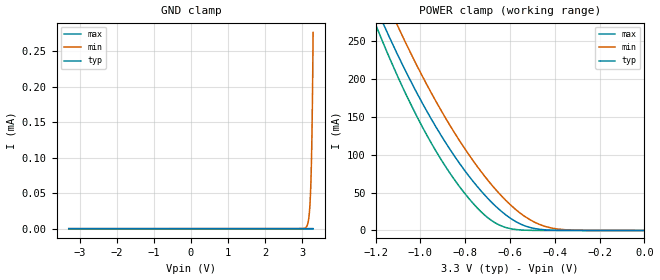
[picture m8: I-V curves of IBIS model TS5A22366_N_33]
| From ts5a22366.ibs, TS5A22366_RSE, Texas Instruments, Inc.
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[Model]   TS5A22366_N_33
Model_type  Terminator
| variable   typ   min   max
C_comp   39.25pF   35.88pF   43.33pF
| C_tri-state   39.25pF   35.88pF   43.33pF
[Temperature Range]   40   100   -40
| Ambient temperature   25   85   -40
[Voltage range]   3.3   3   3.6
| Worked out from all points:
|   POWER clamp passes 1 mA (typ) near -0.45 V on its own axis
[GND Clamp]
| TS5A22366_N_33
|   Voltage   I(typ)   I(min)   I(max)
-3.3V     -900.2pA   -83.56nA   -200.8pA
3.1V      446.7pA    1.439uA    30.69pA
3.15V     455pA      5.868uA    32.16pA
3.185V    463.9pA    15.31uA    33.19pA
3.21V     476.1pA    29.74uA    33.92pA
3.235V    502.8pA    56.7uA     34.65pA
3.255V    549.6pA    93.65uA    35.23pA
3.27V     616.4pA    135.3uA    35.66pA
3.28V     687.6pA    172.2uA    35.95pA
3.285V    734.8pA    194.1uA    36.09pA
3.295V    861.4pA    245.9uA    36.38pA
3.3V      945.5pA    276.5uA    36.52pA
[POWER Clamp]
| TS5A22366_N_33
|   Voltage   I(typ)   I(min)   I(max)
-3.3V     2.809A     2.826A     3.106A
-1.205V   299.6mA    339.7mA    275.9mA
-1.185V   286mA      325.8mA    261.2mA
-1.16V    269.4mA    308.7mA    243.3mA
-1.1V     231.1mA    269.4mA    202.5mA
-990mV    167.6mA    203.1mA    136.1mA
-885mV    114.9mA    147.2mA    83.22mA
-765mV    64.93mA    92.29mA    35.89mA
-670mV    33.75mA    56.18mA    10.79mA
-555mV    8.756mA    23.08mA    727.7uA
-445mV    909uA      5.508mA    18.01uA
0V        0A         0A         0A
